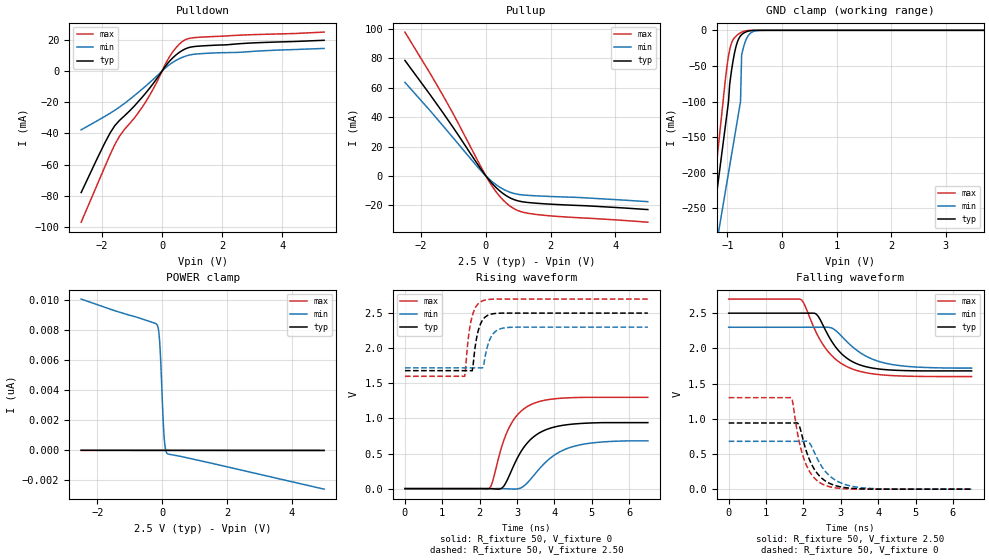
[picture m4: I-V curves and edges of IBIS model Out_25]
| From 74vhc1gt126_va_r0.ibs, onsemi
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|//////////////////////////////////////////////////////////////////////////////
|//////////////////////////////////////////////////////////////////////////////
[Model] Out_25
Model_type 3-state
Polarity Non-Inverting
Enable Active-High
Vmeas = 1.25
Vref = 2.50
Rref = 1k
Cref = 15pF
|  variable   typ   min   max
C_comp   3.8pF   3.8pF   3.8pF
|//////////////////////////////////////////////////////////////////////////////
[Temperature Range]   25   125   -55
|//////////////////////////////////////////////////////////////////////////////
[Voltage Range]   2.50V   2.30V   2.70V
|//////////////////////////////////////////////////////////////////////////////
[Pulldown Reference]   0V   0V   0V
|//////////////////////////////////////////////////////////////////////////////
[Pullup Reference]   2.50V   2.30V   2.70V
|//////////////////////////////////////////////////////////////////////////////
[GND Clamp Reference]   0V   0V   0V
|//////////////////////////////////////////////////////////////////////////////
[POWER Clamp Reference] 2.50V   2.30V   2.70V
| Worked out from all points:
|   slope of the pulldown table from 0 to 0.375 V, typ, clamps not added: 43 ohm
|   slope of the pullup table from 0 to 0.375 V, typ, clamps not added: 40.9 ohm
|   GND clamp passes 1 mA (typ) near -0.61 V on its own axis
|   falling waveform, R_fixture 50, V_fixture 2.50: 20-80 % time 690ps typ, 899ps min, 784ps max; typ from 2.5 V to 1.68 V
|   falling waveform, R_fixture 50, V_fixture 0: 20-80 % time 462ps typ, 558ps min, 387ps max; typ from 0.94 V to 0 V
|   rising waveform, R_fixture 50, V_fixture 0: 20-80 % time 684ps typ, 854ps min, 571ps max; typ from 0 V to 0.94 V
|   rising waveform, R_fixture 50, V_fixture 2.50: 20-80 % time 175ps typ, 200ps min, 174ps max; typ from 1.68 V to 2.5 V
|//////////////////////////////////////////////////////////////////////////////
[Pulldown]
|   Voltage   I(typ)   I(min)   I(max)
-2.7V     -77.77mA   -37.66mA   -96.72mA
-1.92V    -46.36mA   -29.19mA   -61.67mA
-1.58V    -35.04mA   -25.19mA   -47.15mA
-1.26V    -28.78mA   -20.85mA   -37.48mA
-660mV    -16.71mA   -11.53mA   -23.09mA
-280mV    -7.633mA   -5.093mA   -10.92mA
220mV     5.625mA    3.668mA    8.236mA
420mV     9.519mA    6.251mA    13.83mA
660mV     12.92mA    8.558mA    18.53mA
860mV     14.74mA    9.89mA     20.56mA
1.22V     15.84mA    10.94mA    21.49mA
5.4V      19.58mA    14.36mA    24.82mA
|//////////////////////////////////////////////////////////////////////////////
[Pullup]
|   Voltage   I(typ)   I(min)   I(max)
-2.5V     78.63mA    63.73mA    97.94mA
-1.72V    55.24mA    44.36mA    69.74mA
-1.32V    42.83mA    34.01mA    54.6mA
-880mV    28.72mA    22.5mA     36.96mA
-280mV    8.722mA    6.723mA    11.53mA
80mV      -2.248mA   -1.696mA   -3.042mA
240mV     -6.271mA   -4.718mA   -8.513mA
400mV     -9.669mA   -7.254mA   -13.18mA
720mV     -14.63mA   -10.89mA   -20.12mA
1.04V     -17.22mA   -12.69mA   -24.01mA
1.56V     -18.59mA   -13.56mA   -26.25mA
5V        -22.91mA   -17.53mA   -31.49mA
|//////////////////////////////////////////////////////////////////////////////
[GND Clamp]
|   Voltage   I(typ)   I(min)   I(max)
-2.5V     -1.002A    -891.1mA   -1.133A
-1.36V    -325.3mA   -372.7mA   -303.7mA
-1.28V    -277.8mA   -336.3mA   -245.4mA
-1.12V    -182.9mA   -263.6mA   -129mA
-980mV    -99.86mA   -199.9mA   -35.85mA
-960mV    -76.52mA   -190.8mA   -27.68mA
-880mV    -35.51mA   -154.4mA   -11.27mA
-760mV    -7.765mA   -99.87mA   -3.415mA
-740mV    -6.079mA   -34.88mA   -2.596mA
-620mV    -1.172mA   -7.61mA    -163.2uA
-440mV    -8.268uA   -318.2uA   -40.44nA
5V        5.945pA    1.212nA    284.4fA
|//////////////////////////////////////////////////////////////////////////////
[POWER Clamp]
|   Voltage   I(typ)   I(min)   I(max)
-2.5V     5.945pA    10.09nA    292.4fA
-160mV    2.443pA    8.392nA    199fA
-120mV    2.383pA    8.139nA    197.4fA
-80mV     2.323pA    7.358nA    195.8fA
-60mV     2.293pA    6.661nA    195fA
-40mV     2.263pA    5.757nA    194.2fA
20mV      2.174pA    2.531nA    191.8fA
40mV      2.144pA    1.622nA    191fA
60mV      2.114pA    916.2pA    190.2fA
100mV     2.054pA    105.4pA    188.6fA
160mV     1.964pA    -216.9pA   186.2fA
5V        -5.279pA   -2.586nA   -6.904fA
|//////////////////////////////////////////////////////////////////////////////
|//////////////////////////////////////////////////////////////////////////////
[Ramp]
|  variable   typ   min   max
dV/dt_r   5.640E-01/7.000E-10  4.080E-01/8.500E-10  7.800E-01/5.500E-10
dV/dt_f   4.920E-01/7.000E-10  3.480E-01/9.000E-10  6.600E-01/8.000E-10
R_load = 50
|/////////////////////////////////////////////////////////////////////////////
[Falling Waveform]
R_fixture = 50
V_fixture = 2.50
V_fixture_min = 2.30
V_fixture_max = 2.70
C_fixture = 0p
|   time   V(typ)   V(min)   V(max)
0s        2.5V       2.3V       2.7V
1.95ns    2.5V       2.3V       2.689V
2.35ns    2.484V     2.3V       2.217V
2.6ns     2.248V     2.301V     1.996V
2.75ns    2.105V     2.291V     1.901V
2.95ns    1.963V     2.211V     1.809V
3.4ns     1.788V     1.984V     1.69V
3.85ns    1.72V      1.847V     1.639V
4.4ns     1.691V     1.768V     1.613V
6.5ns     1.68V      1.72V      1.6V
|//////////////////////////////////////////////////////////////////////////////
[Falling Waveform]
R_fixture = 50
V_fixture = 0
C_fixture = 0p
|   time   V(typ)   V(min)   V(max)
0s        940mV      680mV      1.3V
1.675ns   939.9mV    680mV      1.299V
1.725ns   939.5mV    680mV      1.2V
1.875ns   917.4mV    679.7mV    705.9mV
2.05ns    586.5mV    682.2mV    377.8mV
2.3ns     276.5mV    514.7mV    153.9mV
2.6ns     111.8mV    244.2mV    51.1mV
2.95ns    37.84mV    101mV      12.56mV
3.5ns     5.237mV    24.03mV    0V
6.5ns     0V         0V         0V
|//////////////////////////////////////////////////////////////////////////////
[Rising Waveform]
R_fixture = 50
V_fixture = 0
C_fixture = 0p
|   time   V(typ)   V(min)   V(max)
0s        0V         0V         0V
2.25ns    1.112mV    -3.687uV   -2.148mV
2.35ns    -2.202mV   16.23uV    108.9mV
2.6ns     9.092mV    668uV      614.3mV
2.8ns     194.5mV    -4.556mV   881.8mV
3.1ns     522.2mV    9.309mV    1.1V
3.45ns    740.4mV    189.3mV    1.215V
3.95ns    870.3mV    458.8mV    1.276V
4.45ns    917mV      591.4mV    1.295V
6.5ns     940mV      680mV      1.3V
|//////////////////////////////////////////////////////////////////////////////
[Rising Waveform]
R_fixture = 50
V_fixture = 2.50
V_fixture_min = 2.30
V_fixture_max = 2.70
C_fixture = 0p
|   time   V(typ)   V(min)   V(max)
0s        1.68V      1.72V      1.6V
1.6ns     1.68V      1.72V      1.599V
1.7ns     1.68V      1.72V      2.159V
1.775ns   1.68V      1.72V      2.402V
1.8ns     1.678V     1.72V      2.456V
1.95ns    2.225V     1.72V      2.627V
2.1ns     2.417V     1.737V     2.679V
2.3ns     2.484V     2.155V     2.697V
2.6ns     2.5V       2.283V     2.7V
6.5ns     2.5V       2.3V       2.7V
